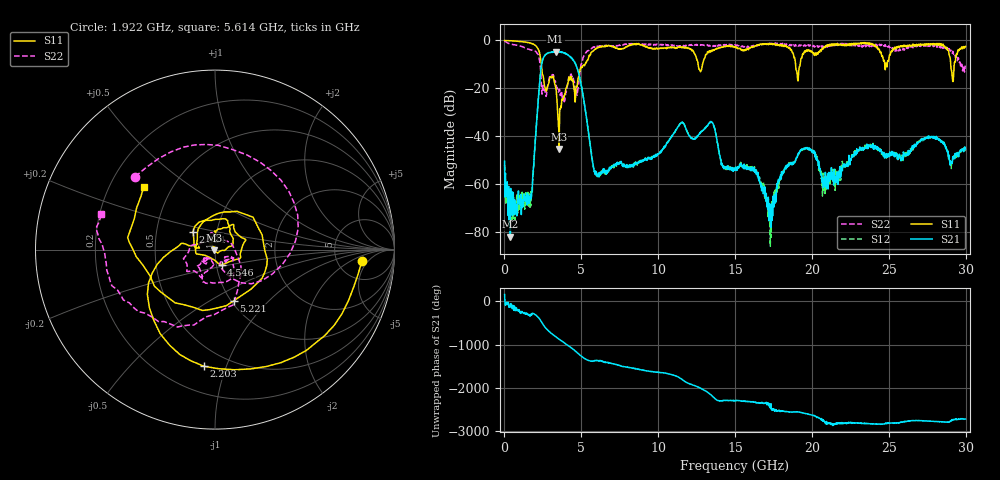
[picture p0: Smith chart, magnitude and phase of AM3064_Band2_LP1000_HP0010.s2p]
# Hz S DB R 50.0
!freq dBS11 angS11 dBS21 angS21 dBS12 angS12 dBS22 angS22
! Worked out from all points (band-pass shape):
!   1600 points, 10 MHz to 29.98 GHz, reference 50 ohm
!   highest |S21| = -4.62 dB at 3.328 GHz (marker M1); lowest = -81.9 dB at 384.9 MHz (marker M2)
!   |S21| within 3 dB of the highest: 2.513 GHz to 4.389 GHz (1.876 GHz wide, 54.4 % of centre)
!   lowest |S11| = -45.3 dB at 3.553 GHz (marker M3), VSWR 1.01, Z = 49.6 - j0.338 ohm
!   |S11| at or under -10 dB: 2.397 GHz to 5.237 GHz (2.839 GHz wide, 74.4 % of centre); 12.6 GHz to 12.88 GHz (283.5 MHz wide, 2.22 % of centre); 18.93 GHz to 19.23 GHz (301.8 MHz wide, 1.58 % of centre)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
!   |S22| runs from -25.6 to -0.2 dB; largest |S21 - S12| = 0.022
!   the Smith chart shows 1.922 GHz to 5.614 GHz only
!   S11 on the Smith chart (normalised r, x): 1.922 GHz: 8.81, -3.47; 2.203 GHz: 0.37, -0.84; 2.934 GHz: 0.77, +0.16; 4.546 GHz: 1.06, -0.18; 5.221 GHz: 1.03, -0.65; 5.614 GHz: 0.35, +0.34
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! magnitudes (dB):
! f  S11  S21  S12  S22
! 10 MHz  0.0  -50.4  -52.0  -0.2
! 384.9 MHz  -0.2  -81.9  -71.3  -1.5
! 1.622 GHz  -1.0  -65.9  -64.6  -3.7
! 1.922 GHz  -1.7  -49.7  -50.0  -4.4
! 2.203 GHz  -3.7  -24.5  -24.5  -6.0
! 2.934 GHz  -16.1  -5.1  -5.1  -15.1
! 3.328 GHz  -19.4  -4.6  -4.7  -17.3
! 3.553 GHz  -45.3  -4.8  -4.8  -20.5
! 4.546 GHz  -20.8  -8.8  -8.8  -17.4
! 5.015 GHz  -11.4  -19.4  -19.3  -9.7
! 5.221 GHz  -10.3  -27.2  -27.2  -5.9
! 5.614 GHz  -5.5  -45.5  -45.1  -3.6
! 6.083 GHz  -3.1  -56.6  -55.4  -2.5
! 10 GHz  -3.4  -47.3  -47.0  -1.8
! 13.43 GHz  -4.5  -33.8  -33.9  -2.4
! 15 GHz  -2.6  -53.8  -53.2  -1.8
! 16.34 GHz  -2.3  -53.8  -54.9  -2.4
! 17.27 GHz  -1.3  -74.6  -79.7  -1.2
! 19.99 GHz  -4.6  -46.0  -45.6  -1.9
! 20.8 GHz  -2.6  -57.6  -57.3  -2.6
! 25 GHz  -8.1  -47.4  -48.5  -2.3
! 29.98 GHz  -2.5  -45.3  -45.9  -10.5
